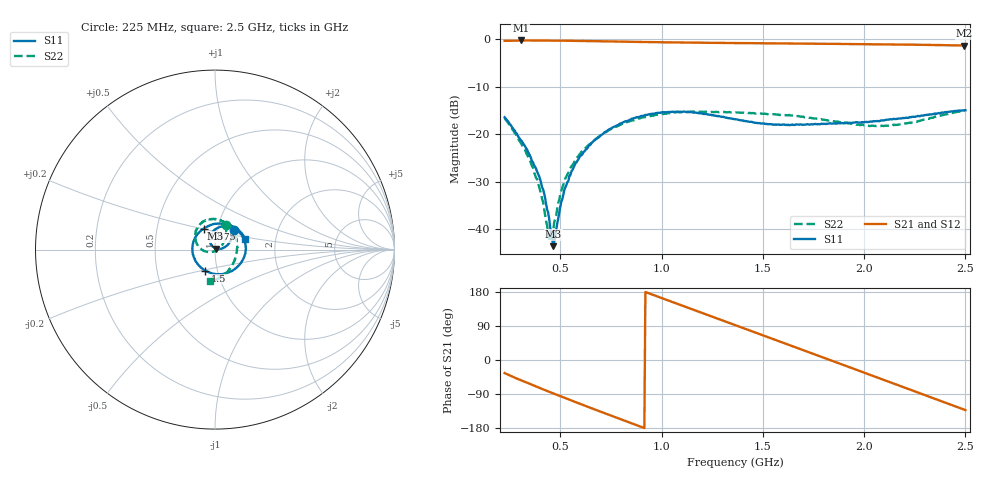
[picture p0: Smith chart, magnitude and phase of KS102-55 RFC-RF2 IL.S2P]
!Agilent	"Technologies,E8364B,MY43040668,A.07.50.67"
!Agilent	E8364B:	A.07.50.67
!Date:	"Tuesday,"	September	"22,"	2015	13:35:53
!Correction:	S11(Full	2	"Port(1,2))"
!S21(Full	2	"Port(1,2))"
!S12(Full	2	"Port(1,2))"
!S22(Full	2	"Port(1,2))"
!S2P	File:	Measurements:	"S11,"	"S21,"	"S12,"	S22:
#	Hz	S	dB	R	50
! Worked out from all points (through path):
!   456 points, 225 MHz to 2.5 GHz, reference 50 ohm
!   highest |S21| = -0.27 dB at 305 MHz (marker M1); lowest = -1.3 dB at 2.495 GHz (marker M2)
!   group delay of S21, straight-line fit = 552 ps
!   lowest |S11| = -43.6 dB at 465 MHz (marker M3), VSWR 1.01, Z = 50.3 + j0.585 ohm
!   |S11| at or under -10 dB: start of sweep to end of sweep
!   |S22| runs from -42.5 to -15.0 dB; largest |S21 - S12| = 0.0043
!   S11 on the Smith chart (normalised r, x): 225 MHz: 1.20, +0.27; 1.5 GHz: 0.87, -0.21; 1.975 GHz: 0.86, +0.20; 2.5 GHz: 1.39, +0.17
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2.25e8  -16.46 46.7  -0.35 -34.5  -0.33 -34.5  -16.59 66.0
3.05e8  -21.29 25.1  -0.27 -53.4  -0.25 -53.4  -21.85 47.3
3.95e8  -28.84 8.2  -0.28 -73.2  -0.26 -73.2  -31.12 19.3
4.45e8  -37.81 21.2  -0.29 -83.9  -0.28 -83.9  -42.07 -51.7
4.65e8  -43.63 61.9  -0.30 -88.1  -0.27 -88.1  -40.45 -105.9
4.75e8  -41.55 89.7  -0.30 -90.2  -0.28 -90.2  -37.90 -124.4
5.2e8  -31.74 128.8  -0.32 -99.6  -0.30 -99.6  -30.03 -153.6
6.05e8  -24.45 119.0  -0.37 -117.2  -0.35 -117.1  -23.68 -173.9
7.95e8  -17.78 78.3  -0.51 -155.7  -0.49 -155.7  -18.08 151.1
8.9e8  -16.37 56.4  -0.58 -174.7  -0.56 -174.6  -16.71 137.0
9.85e8  -15.50 34.0  -0.64 166.6  -0.61 166.6  -15.86 123.7
1.19e9  -15.61 -18.7  -0.74 126.1  -0.72 126.2  -15.30 102.2
1.365e9  -16.87 -70.9  -0.82 91.7  -0.79 91.8  -15.41 87.4
1.5e9  -17.76 -115.3  -0.86 65.2  -0.84 65.2  -15.71 76.5
1.63e9  -18.14 -157.0  -0.91 39.6  -0.88 39.6  -15.96 64.4
1.745e9  -17.98 170.4  -0.95 16.9  -0.93 16.9  -16.66 50.1
1.86e9  -17.81 142.9  -0.98 -5.6  -0.97 -5.6  -17.36 32.1
1.975e9  -17.59 118.7  -1.04 -28.3  -1.02 -28.3  -18.03 10.9
2.125e9  -16.90 92.5  -1.11 -58.1  -1.08 -58.0  -18.23 -23.2
2.305e9  -15.97 59.4  -1.19 -93.6  -1.18 -93.6  -16.90 -63.4
2.495e9  -14.99 20.2  -1.33 -131.2  -1.31 -131.1  -14.99 -98.5
2.5e9  -14.97 18.8  -1.32 -132.1  -1.31 -132.1  -14.96 -99.1
